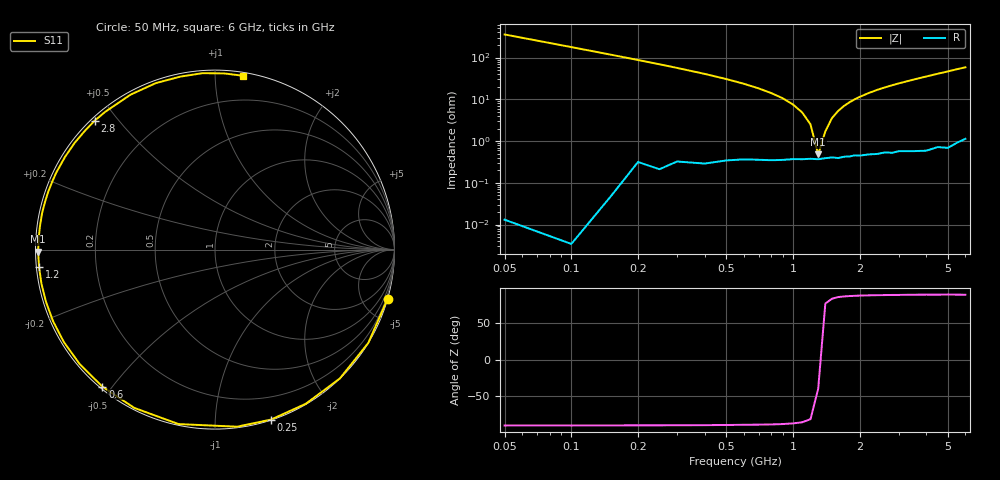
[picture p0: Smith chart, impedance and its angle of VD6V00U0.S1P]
! Infineon Technologies  Discrete & RF Semiconductors
! BBY 55-03
! Si Tuning Diode in SOD323
! VR = 6 V
! S-Parameters:  June  1999
# GHz  S  MA  R  50
!  f  S11
! GHz  MAG  ANG
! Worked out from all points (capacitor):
!   34 points, 50 MHz to 6 GHz, reference 50 ohm
!   read as one part to ground: C = 8.87 pF near 50 MHz
!   lowest |Z| = 478 mohm at 1.3 GHz (marker M1)
!   series resonance near 1.316 GHz, so ESL is about 1.7 nH
!   S11 on the Smith chart (normalised r, x): 50 MHz: 0.00, -7.16; 250 MHz: 0.00, -1.38; 600 MHz: 0.01, -0.47; 1.2 GHz: 0.01, -0.05; 2.8 GHz: 0.01, +0.43; 6 GHz: 0.02, +1.17
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0.05  1 -15.9
0.1  1 -31.3
0.15  0.9997 -45.9
0.2  0.9969 -59.5
0.25  0.9971 -71.8
0.3  0.9943 -82.9
0.4  0.993 -101.8
0.5  0.99 -117.0
0.6  0.9881 -129.4
0.7  0.9875 -139.8
0.8  0.9872 -148.6
0.9  0.9865 -156.1
1  0.9857 -162.9
1.2  0.9851 -174.3
1.3  0.9854 -179.3
1.5  0.9839 171.9
1.6  0.9846 168.0
1.8  0.9835 160.7
2  0.9831 154.2
2.4  0.9825 142.8
2.8  0.9825 133.1
3  0.9816 128.6
3.5  0.9832 118.6
4  0.9844 109.5
4.5  0.9829 101.3
5  0.9854 94.0
5.5  0.9828 87.0
6  0.981 81.0
